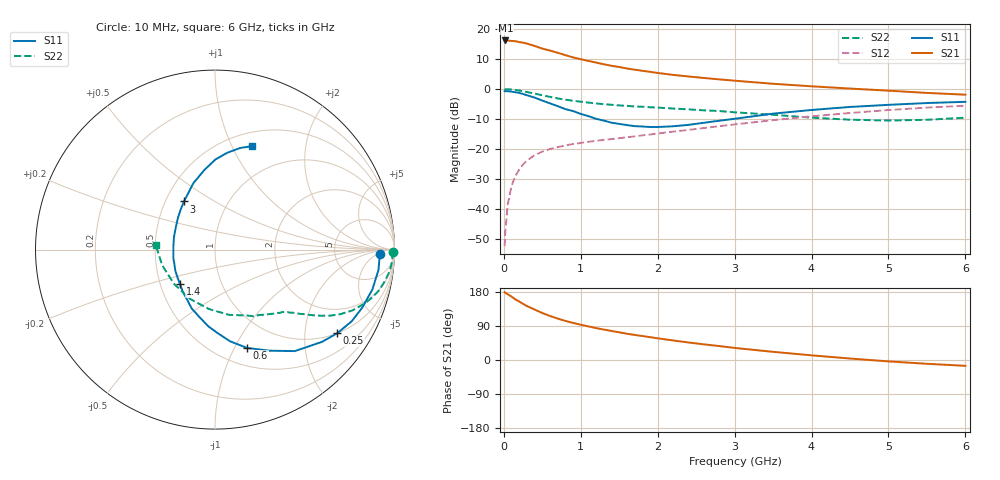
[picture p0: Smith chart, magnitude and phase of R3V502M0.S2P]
! SIEMENS Small Signal Semiconductors
! BFR181
! Si NPN RF Bipolar Junction Transistor in SOT23
! VCE = 0.5 V  IC = 2 mA
! Common Emitter S-Parameters:  May  1996
# GHz  S  MA  R  50
!  f  S11  S21  S12  S22
! GHz  MAG  ANG  MAG  ANG  MAG  ANG  MAG  ANG
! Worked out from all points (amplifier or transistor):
!   36 points, 10 MHz to 6 GHz, reference 50 ohm
!   highest |S21| = 16.2 dB at 20 MHz (marker M1)
!   |S21| within 3 dB of that: start of sweep to 542.9 MHz
!   unconditionally stable (mu >= 1): 1.36 GHz to 4.17 GHz
!   at 250 MHz: K = 0.26, MSG = 20.3 dB, |S12| = -25.1 dB
!   at 1.4 GHz: K = 1.02, MAG = 11.4 dB, |S12| = -16.7 dB
!   at 6 GHz: K = 0.95, MSG = 1.8 dB, |S12| = -5.6 dB
!   S11 on the Smith chart (normalised r, x): 10 MHz: 22, -8; 250 MHz: 1.00, -2.92; 600 MHz: 0.69, -1.13; 1.4 GHz: 0.63, -0.26; 3 GHz: 0.62, +0.37; 6 GHz: 0.65, +1.19
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0.01  0.9219 -1.6  6.394 178.9  0.0024 90.0  0.9932 -0.8
0.02  0.918 -2.8  6.442 177.2  0.0044 83.8  0.9886 -1.5
0.05  0.9179 -7.1  6.401 173.5  0.0117 84.6  0.989 -3.7
0.1  0.9046 -14.2  6.329 167.3  0.0243 81.0  0.9806 -7.1
0.15  0.8822 -21.4  6.258 159.9  0.0355 77.0  0.9607 -10.8
0.25  0.8252 -34.4  5.918 148.1  0.0553 69.5  0.9177 -16.7
0.3  0.7868 -40.8  5.71 142.3  0.064 66.7  0.8901 -19.5
0.4  0.7196 -51.8  5.216 133.2  0.0788 61.2  0.8374 -23.9
0.5  0.6404 -61.6  4.714 124.0  0.0904 57.1  0.7862 -27.2
0.6  0.5765 -71.9  4.364 116.1  0.1001 53.7  0.7388 -29.9
0.7  0.5176 -80.7  4.017 109.3  0.1074 51.4  0.6974 -31.9
0.8  0.4623 -88.7  3.663 103.1  0.1143 49.6  0.6637 -33.5
0.9  0.429 -95.0  3.365 97.9  0.1211 48.5  0.6367 -34.8
1.1  0.3523 -111.7  2.937 88.6  0.1317 47.0  0.5932 -37.1
1.4  0.2742 -135.3  2.435 76.6  0.1465 46.6  0.5455 -40.1
1.7  0.2405 -160.0  2.099 66.2  0.162 47.4  0.5117 -42.8
2.2  0.239 163.1  1.718 51.6  0.1944 48.0  0.4723 -49.4
3  0.3189 122.8  1.375 31.9  0.2567 46.5  0.4088 -64.0
3.5  0.3884 108.2  1.222 21.5  0.3026 43.7  0.3717 -77.9
4.5  0.5019 89.8  1.017 3.9  0.3982 34.4  0.3078 -117.3
5.5  0.5832 76.1  0.86 -10.0  0.4892 22.2  0.3069 -163.7
6  0.6114 70.5  0.804 -15.4  0.5274 15.4  0.3322 175.2
